| TEXAS INSTRUMENTS INCORPORATED
| Standard Linear and Logic Group
| IBIS Model of SN74LVTH244A
| 3.3-V ABT OCTAL BUFFERS/DRIVERS WITH 3-STATE OUTPUTS
| This file contains package information for the following:
|  TSSOP 20-pin (PW) package as [Component] LVTH244A_PW
|  SOIC 20-pin (DW) package as [Component] LVTH244A_DW
|  SOP 20-pin (NS) package as [Component] LVTH244A_NS
|  SSOP 20-pin (DB) package as [Component] LVTH244A_DB
|  VFBGA 20-pin (GQN) package as [Component] LVTH244A_GQN
| This device can be powered at the following Vccs:
|  2.8 volt Vcc
|  3.3 volt Vcc
| This file provides unique models under the [Model Selector] for each Vcc.
| For operation at a specific Vcc, select the appropriate model after each
| [Model Selector] keyword.
[IBIS Ver]   3.2
[Comment char]  |_char
[File Name]   sn74lvth244a.ibs
[File Rev]   1.1 | a_die
[Date]   April 18, 2002
[Source]   Data created from TI-SPICE simulations at TI-SLL.
[Notes]   The following is an IBIS list for the SN74LVTH244A.
   Please contact sllibis@ti.com with questions and
   comments concerning SLL IBIS models.
   -NON MONOTONIC DATA IN PULLUP AS THE DEVICE IS OVERVOLTAGE
   TOLERANT
   -NON MONOTONIC DATA IN GND CLAMP DUE TO BUS HOLD CIRCUIT
   -Power clamp data deleted as there is no power-clamp diode.
[Disclaimer] Property of Texas Instruments Incorporated.  Unauthorized
   reproduction and/or distribution is strictly prohibited.
   This product is protected under copyright law.
   Created  2002, (C) Copyright  2002, Texas Instruments
   Incorporated, All Rights Reserved
   UNLESS THERE IS A SIGNED, WRITTEN AGREEMENT TO THE
   CONTRARY, TEXAS INSTRUMENTS (TI) IS PROVIDING THE IBIS
   MODELS  AND WITHOUT ANY WARRANTY, EXPRESSED OR
   IMPLIED.  TI assumes no liability for:
   1) the accuracy of the IBIS models provided to your
   company;
   2) the proper functioning of these IBIS Models in your
   design or for any resulting applications; or
   3) infringement of patents, copyrights or intellectual
   property rights resulting from your use of these IBIS
   models.
   TI provides IBIS Models as a service to our customers.
   You and your company shall not distribute, sell or give
   these models to anyone else without prior written
   permission from TI.
   TI reserves the right to make changes to our products or
   to discontinue any semiconductor product or service
   without notice, and advises our customers to obtain the
   latest version of relevant information to verify, before
   placing orders, that the information being relied on is
   current.
   Please be aware that your receipt and use of the IBIS
   information provided shall serve as acceptance of these
   terms and conditions.  If you do not accept these terms,
   you should return or destroy the IBIS models and any
   other accompanying information immediately.
| Component LVTH244A_PW 20-pin TSSOP
[Component]   LVTH244A_PW
[Manufacturer]   Texas Instruments, Inc.
[Package]
|   typ   min   max
R_pkg   4.500e-02   3.600e-02   5.700e-02
L_pkg   2.694e-09   2.290e-09   3.177e-09
C_pkg   1.560e-13   7.600e-14   2.590e-13
[Pin]   signal_name  model_name   R_pin   L_pin   C_pin
1   1NOE   LVTH244A_OE   3.600e-02   3.045e-09   2.590e-13
2   1A1   LVTH244A_IN   5.100e-02   3.013e-09   1.890e-13
3   2Y4   LVTH244A_OUT   4.400e-02   2.695e-09   1.640e-13
4   1A2   LVTH244A_IN   4.700e-02   2.362e-09   7.900e-14
5   2Y3   LVTH244A_OUT   4.700e-02   2.333e-09   8.600e-14
6   1A3   LVTH244A_IN   4.700e-02   2.298e-09   8.500e-14
7   2Y2   LVTH244A_OUT   4.700e-02   2.351e-09   7.900e-14
8   1A4   LVTH244A_IN   4.400e-02   2.706e-09   1.650e-13
9   2Y1   LVTH244A_OUT   4.900e-02   2.999e-09   1.880e-13
10   GND   GND   3.900e-02   3.039e-09   2.570e-13
11   2A1   LVTH244A_IN   3.800e-02   3.044e-09   2.580e-13
12   1Y4   LVTH244A_OUT   5.700e-02   3.177e-09   1.990e-13
13   2A2   LVTH244A_IN   4.400e-02   2.825e-09   1.730e-13
14   1Y3   LVTH244A_OUT   4.700e-02   2.429e-09   8.300e-14
15   2A3   LVTH244A_IN   4.900e-02   2.383e-09   9.000e-14
16   1Y2   LVTH244A_OUT   4.900e-02   2.347e-09   8.900e-14
17   2A4   LVTH244A_IN   4.700e-02   2.290e-09   7.600e-14
18   1Y1   LVTH244A_OUT   4.500e-02   2.613e-09   1.580e-13
19   2NOE   LVTH244A_OE   4.400e-02   2.883e-09   1.810e-13
20   VCC   POWER   3.900e-02   3.044e-09   2.560e-13
| Component LVTH244A_DW 20-pin SOIC
[Component]   LVTH244A_DW
[Manufacturer]  Texas Instruments, Inc.
[Package]
|   typ   min   max
R_pkg   3.800e-02   3.300e-02   4.500e-02
L_pkg   5.012e-09   4.110e-09   6.349e-09
C_pkg   7.170e-13   5.300e-13   8.680e-13
[Pin]   signal_name  model_name   R_pin   L_pin   C_pin
1   1NOE   LVTH244A_OE   4.200e-02   6.336e-09   8.650e-13
2   1A1   LVTH244A_IN   4.300e-02   5.542e-09   8.670e-13
3   2Y4   LVTH244A_OUT   3.400e-02   4.714e-09   7.320e-13
4   1A2   LVTH244A_IN   3.400e-02   4.377e-09   5.910e-13
5   2Y3   LVTH244A_OUT   3.600e-02   4.130e-09   5.330e-13
6   1A3   LVTH244A_IN   3.500e-02   4.111e-09   5.300e-13
7   2Y2   LVTH244A_OUT   3.400e-02   4.284e-09   5.830e-13
8   1A4   LVTH244A_IN   3.400e-02   4.634e-09   7.260e-13
9   2Y1   LVTH244A_OUT   4.000e-02   5.518e-09   8.650e-13
10   GND   GND   4.300e-02   6.349e-09   8.660e-13
11   2A1   LVTH244A_IN   4.100e-02   6.281e-09   8.610e-13
12   1Y4   LVTH244A_OUT   4.500e-02   5.561e-09   8.680e-13
13   2A2   LVTH244A_IN   3.300e-02   4.778e-09   7.420e-13
14   1Y3   LVTH244A_OUT   3.500e-02   4.414e-09   5.960e-13
15   2A3   LVTH244A_IN   3.500e-02   4.110e-09   5.330e-13
16   1Y2   LVTH244A_OUT   3.600e-02   4.130e-09   5.330e-13
17   2A4   LVTH244A_IN   3.400e-02   4.377e-09   5.910e-13
18   1Y1   LVTH244A_OUT   3.400e-02   4.714e-09   7.310e-13
19   2NOE   LVTH244A_OE   4.300e-02   5.569e-09   8.680e-13
20   VCC   POWER   4.200e-02   6.308e-09   8.640e-13
| Component LVTH244A_NS 20-pin SOP
[Component]   LVTH244A_NS
[Manufacturer]  Texas Instruments, Inc.
[Package]
|   typ   min   max
R_pkg   4.400e-02   2.900e-02   5.800e-02
L_pkg   3.666e-09   2.317e-09   5.115e-09
C_pkg   5.480e-13   3.160e-13   7.250e-13
[Pin]   signal_name  model_name   R_pin   L_pin   C_pin
1   1NOE   LVTH244A_OE   5.800e-02   5.115e-09   7.250e-13
2   1A1   LVTH244A_IN   5.300e-02   4.591e-09   7.240e-13
3   2Y4   LVTH244A_OUT   4.900e-02   3.754e-09   5.720e-13
4   1A2   LVTH244A_IN   2.900e-02   2.549e-09   3.880e-13
5   2Y3   LVTH244A_OUT   3.100e-02   2.317e-09   3.160e-13
6   1A3   LVTH244A_IN   3.100e-02   2.317e-09   3.160e-13
7   2Y2   LVTH244A_OUT   2.900e-02   2.556e-09   3.990e-13
8   1A4   LVTH244A_IN   4.900e-02   3.754e-09   5.790e-13
9   2Y1   LVTH244A_OUT   5.300e-02   4.591e-09   7.240e-13
10   GND   GND   5.800e-02   5.115e-09   7.250e-13
11   2A1   LVTH244A_IN   5.800e-02   5.115e-09   7.250e-13
12   1Y4   LVTH244A_OUT   5.300e-02   4.591e-09   7.240e-13
13   2A2   LVTH244A_IN   4.900e-02   3.754e-09   5.790e-13
14   1Y3   LVTH244A_OUT   2.900e-02   2.557e-09   3.990e-13
15   2A3   LVTH244A_IN   3.100e-02   2.317e-09   3.160e-13
16   1Y2   LVTH244A_OUT   3.100e-02   2.317e-09   3.160e-13
17   2A4   LVTH244A_IN   2.900e-02   2.557e-09   3.990e-13
18   1Y1   LVTH244A_OUT   4.900e-02   3.754e-09   5.790e-13
19   2NOE   LVTH244A_OE   5.300e-02   4.591e-09   7.240e-13
20   VCC   POWER   5.800e-02   5.115e-09   7.250e-13
| Component LVTH244A_DB 20-pin SSOP
[Component]   LVTH244A_DB
[Manufacturer] Texas Instruments, Inc.
[Package]
|   typ   min   max
R_pkg   4.000e-02   3.500e-02   5.100e-02
L_pkg   3.495e-09   3.035e-09   4.314e-09
C_pkg   4.200e-13   3.460e-13   5.020e-13
[Pin]   signal_name  model_name   R_pin   L_pin   C_pin
1   1NOE   LVTH244A_OE   4.900e-02   4.310e-09   5.020e-13
2   1A1   LVTH244A_IN   4.800e-02   3.903e-09   4.870e-13
3   2Y4   LVTH244A_OUT   3.500e-02   3.189e-09   3.960e-13
4   1A2   LVTH244A_IN   3.500e-02   3.036e-09   3.470e-13
5   2Y3   LVTH244A_OUT   3.500e-02   3.035e-09   3.670e-13
6   1A3   LVTH244A_IN   3.500e-02   3.035e-09   3.670e-13
7   2Y2   LVTH244A_OUT   3.500e-02   3.036e-09   3.470e-13
8   1A4   LVTH244A_IN   3.500e-02   3.189e-09   3.970e-13
9   2Y1   LVTH244A_OUT   4.700e-02   3.899e-09   4.880e-13
10   GND   GND   5.100e-02   4.314e-09   5.000e-13
11   2A1   LVTH244A_IN   5.100e-02   4.314e-09   5.000e-13
12   1Y4   LVTH244A_OUT   4.700e-02   3.899e-09   4.880e-13
13   2A2   LVTH244A_IN   3.500e-02   3.189e-09   3.970e-13
14   1Y3   LVTH244A_OUT   3.500e-02   3.036e-09   3.460e-13
15   2A3   LVTH244A_IN   3.500e-02   3.035e-09   3.670e-13
16   1Y2   LVTH244A_OUT   3.500e-02   3.035e-09   3.670e-13
17   2A4   LVTH244A_IN   3.500e-02   3.036e-09   3.460e-13
18   1Y1   LVTH244A_OUT   3.500e-02   3.189e-09   3.970e-13
19   2NOE   LVTH244A_OE   4.700e-02   3.899e-09   4.880e-13
20   VCC   POWER   5.100e-02   4.314e-09   5.020e-13
| Component LVTH244A_GQN 20-pin VFBGA
[Component]   LVTH244A_GQN
[Manufacturer]  Texas Instruments, Inc.
[Package]
|   typ   min   max
R_pkg   4.300e-02   3.300e-02   6.100e-02
L_pkg   1.317e-09   8.960e-10   2.088e-09
C_pkg   1.130e-13   6.400e-14   1.900e-13
[Pin]   signal_name  model_name   R_pin   L_pin   C_pin
A2   1NOE   LVTH244A_OE   3.800e-02   1.199e-09   1.210e-13
A1   1A1   LVTH244A_IN   4.000e-02   1.067e-09   1.020e-13
B3   2Y4   LVTH244A_OUT   6.100e-02   1.999e-09   1.900e-13
B1   1A2   LVTH244A_IN   3.300e-02   9.630e-10   7.100e-14
C2   2Y3   LVTH244A_OUT   4.900e-02   1.523e-09   1.230e-13
C1   1A3   LVTH244A_IN   3.300e-02   8.960e-10   6.400e-14
D3   2Y2   LVTH244A_OUT   6.100e-02   1.899e-09   1.640e-13
D1   1A4   LVTH244A_IN   3.300e-02   8.980e-10   6.700e-14
E2   2Y1   LVTH244A_OUT   4.900e-02   1.514e-09   1.280e-13
E1   GND   GND   3.600e-02   1.006e-09   9.400e-14
E3   2A1   LVTH244A_IN   4.900e-02   1.683e-09   1.460e-13
E4   1Y4   LVTH244A_OUT   3.300e-02   1.121e-09   8.900e-14
D2   2A2   LVTH244A_IN   6.100e-02   2.088e-09   1.730e-13
D4   1Y3   LVTH244A_OUT   3.300e-02   1.027e-09   7.100e-14
C3   2A3   LVTH244A_IN   4.900e-02   1.558e-09   1.240e-13
C4   1Y2   LVTH244A_OUT   3.300e-02   9.280e-10   6.700e-14
B2   2A4   LVTH244A_IN   6.100e-02   1.921e-09   1.770e-13
B4   1Y1   LVTH244A_OUT   3.300e-02   9.010e-10   7.700e-14
A4   2NOE   LVTH244A_OE   3.700e-02   9.900e-10   9.800e-14
A3   VCC   POWER   3.500e-02   1.168e-09   1.190e-13
| Model LVTH244A_OE
[Model Selector]   LVTH244A_OE
LVTH244A_OE_28   2.8 volt Vcc
LVTH244A_OE_33   3.3 volt Vcc
| Model LVTH244A_IN
[Model Selector]   LVTH244A_IN
LVTH244A_IN_28   2.8 volt Vcc
LVTH244A_IN_33   3.3 volt Vcc
| Model LVTH244A_OUT
[Model Selector]   LVTH244A_OUT
LVTH244A_OUT_28   2.8 volt Vcc
LVTH244A_OUT_33   3.3 volt Vcc
| Models and submodels in the file (6): LVTH244A_OE_28 (Input), LVTH244A_OE_33 (Input), LVTH244A_IN_28 (Input), LVTH244A_IN_33 (Input), LVTH244A_OUT_28 (3-state), LVTH244A_OUT_33 (3-state)
